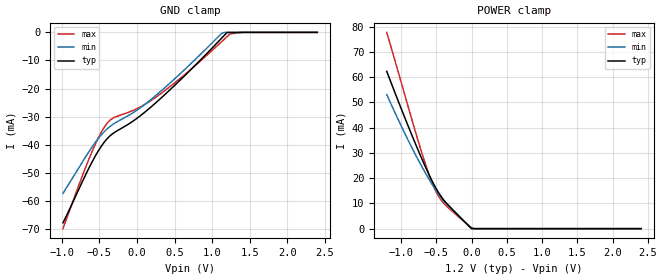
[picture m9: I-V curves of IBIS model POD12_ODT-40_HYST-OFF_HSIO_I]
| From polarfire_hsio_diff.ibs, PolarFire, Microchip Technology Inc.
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|   Model POD12_ODT-40_HYST-OFF_HSIO_I
[Model]   POD12_ODT-40_HYST-OFF_HSIO_I
Model_type   Input
Vinl =   0.76
Vinh =   0.92
|   typ   min   max
C_comp_pullup   1.335e-12   1.335e-12   1.380e-12
C_comp_pulldown  1.335e-12   1.335e-12   1.380e-12
[Temperature Range]  25C   100C   -40C
[Voltage Range]  1.2   1.14   1.26
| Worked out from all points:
|   POWER clamp passes 1 mA (typ) near -0.04 V on its own axis
[GND Clamp]
| Voltage   I(typ)   I(min)   I(max)
-984.4mV  -67.85mA   -57.37mA   -69.94mA
-590.6mV  -45.82mA   -40.58mA   -42.03mA
-472.5mV  -40.48mA   -36.46mA   -35.45mA
-354.4mV  -36.76mA   -33.42mA   -31.19mA
0V        -30.62mA   -27.7mA    -27.17mA
262.5mV   -24.8mA    -22.22mA   -22.89mA
637.5mV   -15.37mA   -13.17mA   -14.97mA
1.125V    -2.11mA    -403.9uA   -3.375mA
1.2V      474.1nA    0A         -1.507mA
1.239V    0A         0A         -518.9uA
1.397V    0A         0A         0A
2.4V      0A         0A         0A
[POWER Clamp]
| Voltage   I(typ)   I(min)   I(max)
-1.2V     62.25mA    53.06mA    77.68mA
-945mV    43.95mA    37.74mA    52.98mA
-748.1mV  30.58mA    26.9mA     34.07mA
-630mV    23.07mA    20.95mA    23.67mA
-551.3mV  18.5mA     17.26mA    17.69mA
-472.5mV  14.51mA    13.9mA     13.07mA
-393.7mV  11.36mA    11mA       10.05mA
-196.9mV  5.557mA    5.331mA    4.954mA
0V        0A         243.8uA    451.3uA
37.5mV    0A         0A         0A
2.4V      0A         0A         0A
